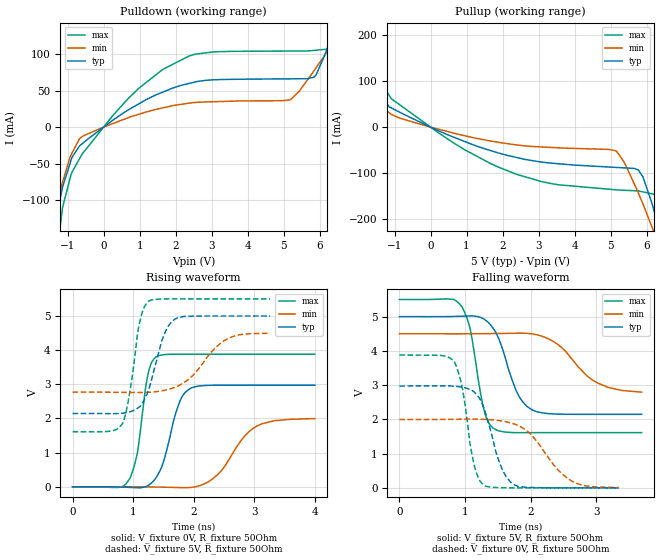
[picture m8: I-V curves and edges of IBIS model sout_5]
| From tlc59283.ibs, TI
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|   sout_5 Model
[Model]   sout_5
Model_type   Output
Polarity   Non-Inverting
Vmeas = 2.5
Vref = 2.5
Cref = 15pF
Rref = 50
|   typ   min   max
 C_comp   1.219e-12   1.129e-12   1.384e-12
| Where nom  PVT is Nominal Process, 5V, 27C
|   Fast PVT is Strong Process,  5.5V, -40C
|   Slow PVT is Weak Process,   4.5V, 125C
[Voltage Range]   5   4.5   5.5
|Ambient Temperature   25   85   -40
|Junction Temperature
[Temperature Range]   27   125   -40
[Pullup Reference]   5   4.5   5.5
[Pulldown Reference]   0   0   0
[Power Clamp Reference]   5   4.5   5.5
[GND Clamp Reference]   0   0   0
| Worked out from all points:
|   slope of the pulldown table from 0 to 0.75 V, typ, clamps not added: 29.6 ohm
|   slope of the pullup table from 0 to 0.75 V, typ, clamps not added: 29.7 ohm
|   falling waveform, V_fixture 5V, R_fixture 50Ohm: 20-80 % time 314ps typ, 522ps min, 207ps max; typ from 5 V to 2.15 V
|   rising waveform, V_fixture 0V, R_fixture 50Ohm: 20-80 % time 272ps typ, 485ps min, 183ps max; typ from 0 V to 2.97 V
|   rising waveform, V_fixture 5V, R_fixture 50Ohm: 20-80 % time 276ps typ, 516ps min, 192ps max; typ from 2.15 V to 5 V
|   falling waveform, V_fixture 0V, R_fixture 50Ohm: 20-80 % time 278ps typ, 501ps min, 190ps max; typ from 2.97 V to 0 V
[Pulldown]
|   Voltage   I(typ)   I(min)   I(max)
-5V       -1.175A    -875.6mA   -1.617A
-1.92V    -292mA     -222.8mA   -452.2mA
-1.373V   -138.4mA   -113.6mA   -201.7mA
-1.14V    -81.73mA   -75.25mA   -109.8mA
-670mV    -25.72mA   -15.92mA   -43.23mA
968mV     31.49mA    17.37mA    52.69mA
2.376V    59.74mA    32.77mA    97.26mA
5.189V    66.01mA    37.33mA    104.1mA
5.85V     68.48mA    77.49mA    105mA
6.418V    135.8mA    118.5mA    107.7mA
6.835V    193.1mA    148.5mA    207.1mA
10V       567.6mA    367.8mA    890.7mA
[Pullup]
|   Voltage   I(typ)   I(min)   I(max)
-5V       500.3mA    295.4mA    839.4mA
-4.004V   397.6mA    229.6mA    718mA
-2.332V   192.2mA    113mA      387.3mA
-1.14V    43.69mA    30.8mA     67.92mA
968mV     -31.98mA   -19.15mA   -50.18mA
3.08V     -76.06mA   -43.22mA   -118.6mA
5.152V    -87.78mA   -51.7mA    -136.5mA
5.775V    -93.52mA   -144.1mA   -138.9mA
6.13V     -161mA     -213.3mA   -144.8mA
6.418V    -238.4mA   -271.1mA   -157.4mA
6.6V      -289.3mA   -307.5mA   -216.8mA
10V       -1.272A    -1.039A    -1.611A
[Ramp]
R_load = 50
|   typ   min   max
dV/dt_r   1.78388/2.70272e-10   1.19731/4.83374e-10   2.32784/1.82223e-10
dV/dt_f   1.71188/3.1345e-10   1.03738/5.32409e-10   2.33259/2.05872e-10
[Falling Waveform]
V_fixture = 5V
V_fixture_min = 4.5V
V_fixture_max = 5.5V
R_fixture = 50Ohm
|   Time   V(typ)   V(min)   V(max)
0s        5V         4.5V       5.5V
950ps     5.012V     4.499V     5.297V
1.07ns    5.02V      4.5V       4.719V
1.3ns     4.915V     4.503V     2.205V
1.43ns    4.659V     4.506V     1.741V
1.775ns   2.863V     4.516V     1.613V
2.02ns    2.284V     4.498V     1.611V
2.425ns   2.153V     4.175V     1.612V
3.01ns    2.147V     3.073V     1.612V
3.695ns   2.147V     2.795V     1.612V
[Rising Waveform]
V_fixture = 0V
V_fixture_min = 0V
V_fixture_max = 0V
R_fixture = 50Ohm
|   Time   V(typ)   V(min)   V(max)
0s        1.601nV    8.788nV    1.176nV
935ps     -16.77mV   779.9uV    214.5mV
1.07ns    -27.6mV    -208.5uV   988.4mV
1.255ns   44.77mV    -3.778mV   3.369V
1.365ns   233mV      -6.706mV   3.785V
1.775ns   2.52V      -23.37mV   3.881V
1.92ns    2.852V     -22.11mV   3.88V
2.39ns    2.973V     349.1mV    3.88V
3.045ns   2.973V     1.78V      3.88V
3.998ns   2.973V     1.996V     3.88V
[Rising Waveform]
V_fixture = 5V
V_fixture_min = 4.5V
V_fixture_max = 5.5V
R_fixture = 50Ohm
|   Time   V(typ)   V(min)   V(max)
0s        2.147V     2.771V     1.613V
630ps     2.141V     2.769V     1.628V
830ps     2.156V     2.765V     1.864V
940ps     2.193V     2.762V     2.721V
1.11ns    2.348V     2.76V      4.829V
1.255ns   2.84V      2.766V     5.429V
1.47ns    4.26V      2.808V     5.496V
1.685ns   4.901V     2.911V     5.501V
2.505ns   5V         4.279V     5.5V
3.26ns    5V         4.495V     5.5V
[Falling Waveform]
V_fixture = 0V
V_fixture_min = 0V
V_fixture_max = 0V
R_fixture = 50Ohm
|   Time   V(typ)   V(min)   V(max)
0s        2.973V     1.996V     3.879V
830ps     2.969V     2.002V     3.71V
950ps     2.941V     2.005V     3.004V
1.14ns    2.797V     2.007V     668.5mV
1.295ns   2.291V     2V         68.41mV
1.54ns    669.3mV    1.959V     5.187mV
1.74ns    102mV      1.872V     -223.3uV
2.02ns    9.607mV    1.53V      -181.2uV
2.645ns   -58.71uV   181.3mV    28.23uV
3.345ns   41.64uV    6.8mV      17.88uV
